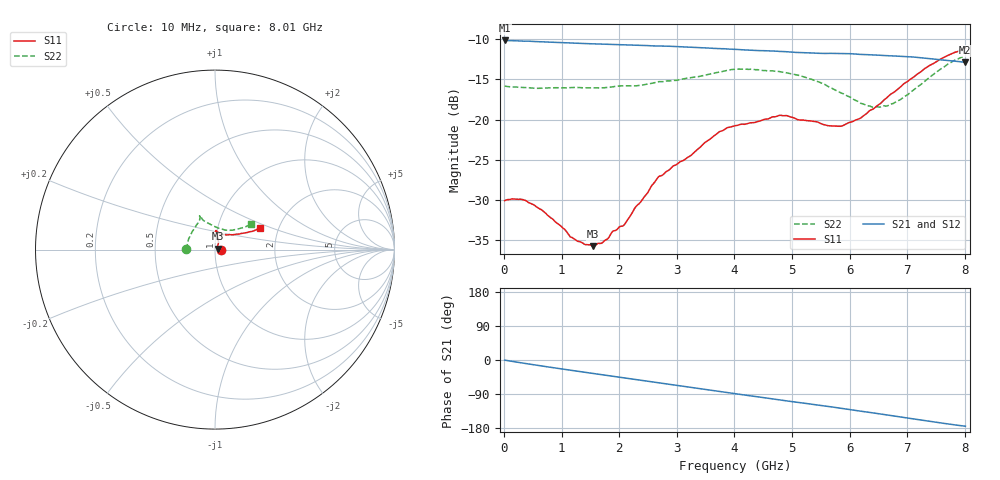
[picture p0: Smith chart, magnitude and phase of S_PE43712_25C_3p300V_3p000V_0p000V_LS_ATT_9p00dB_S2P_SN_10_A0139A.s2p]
! DEVICE ID: PE43712
! File Path: z:\PE43713\PE43713_CHAR_NOM_04292014\AMB\3p300\LS_ATT_9p00dB\PE43713_AMB_3p300V_3p000V_0p000V_LS_ATT_9p00dB_S2P_SN_10_A0139A.s2p
! Serial: 10
! Lot: A0139A
! Temp: 25C
! VDD: 3.300
! VSS: 0.000
! Control_Hi: 3.000
! Control_Lo: 0.000
! Attenuation Step: 9.00dB
! Port 1: RF1
! Port 2: RF2
! ThroughPath:1-2
! IDD: 0.0001469591
! ISS: -4.73e-008
#  Hz  S  RI  R  50
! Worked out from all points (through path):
!   801 points, 10 MHz to 8.01 GHz, reference 50 ohm
!   highest |S21| = -10.15 dB at 10 MHz (marker M1); lowest = -12.9 dB at 8 GHz (marker M2)
!   group delay of S21, straight-line fit = 60 ps
!   lowest |S11| = -35.7 dB at 1.54 GHz (marker M3), VSWR 1.03, Z = 51.6 + j0.477 ohm
!   |S11| at or under -10 dB: start of sweep to end of sweep
!   |S22| runs from -18.5 to -12.1 dB; largest |S21 - S12| = 0.0011
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1e7  0.0313 0.000122  0.3109 -0.00173  0.311 -0.00169  -0.1618 0.00105
3e8  0.0317 -0.00372  0.306 -0.0402  0.306 -0.0402  -0.158 0.0156
5e8  0.0293 -0.00498  0.2997 -0.065  0.2998 -0.0649  -0.1553 0.0247
1.17e9  0.0185 -0.000939  0.2658 -0.1373  0.2659 -0.1375  -0.1476 0.0576
1.35e9  0.0172 0.00117  0.2547 -0.1545  0.2547 -0.1545  -0.144 0.0652
1.54e9  0.0157 0.00462  0.2416 -0.1715  0.2416 -0.1716  -0.1383 0.0751
1.72e9  0.015 0.00856  0.2283 -0.1867  0.2284 -0.1867  -0.1338 0.0838
2.09e9  0.0141 0.0172  0.1981 -0.215  0.1981 -0.2149  -0.1259 0.1024
2.68e9  0.0196 0.0395  0.1429 -0.2489  0.1428 -0.249  -0.1022 0.1386
3.24e9  0.0159 0.0576  0.085 -0.2691  0.0851 -0.2691  -0.0898 0.1588
3.72e9  0.014 0.0819  0.035 -0.2746  0.0347 -0.2746  -0.0839 0.1784
4.01e9  0.0106 0.091  0.00486 -0.2738  0.00483 -0.2738  -0.0858 0.187
4.79e9  0.00518 0.1063  -0.0704 -0.2562  -0.0705 -0.2565  -0.0794 0.1822
5.35e9  0.0154 0.0966  -0.1176 -0.2318  -0.1175 -0.2317  -0.0672 0.1646
5.88e9  0.0383 0.0833  -0.1592 -0.2029  -0.1588 -0.203  -0.029 0.1426
6.38e9  0.0794 0.0835  -0.1909 -0.1656  -0.1906 -0.1657  0.0222 0.1182
6.68e9  0.1124 0.0845  -0.2064 -0.1405  -0.206 -0.1406  0.0577 0.1085
6.99e9  0.1461 0.0897  -0.2193 -0.1128  -0.2189 -0.1128  0.0914 0.1079
7.35e9  0.1887 0.0984  -0.2273 -0.0783  -0.2271 -0.0783  0.1353 0.1171
7.72e9  0.2273 0.1095  -0.2289 -0.0445  -0.2287 -0.0447  0.1798 0.132
8e9  0.2505 0.121  -0.2262 -0.0216  -0.226 -0.0219  0.2021 0.1415
8.01e9  0.2512 0.1218  -0.2263 -0.021  -0.226 -0.0214  0.2027 0.1417
